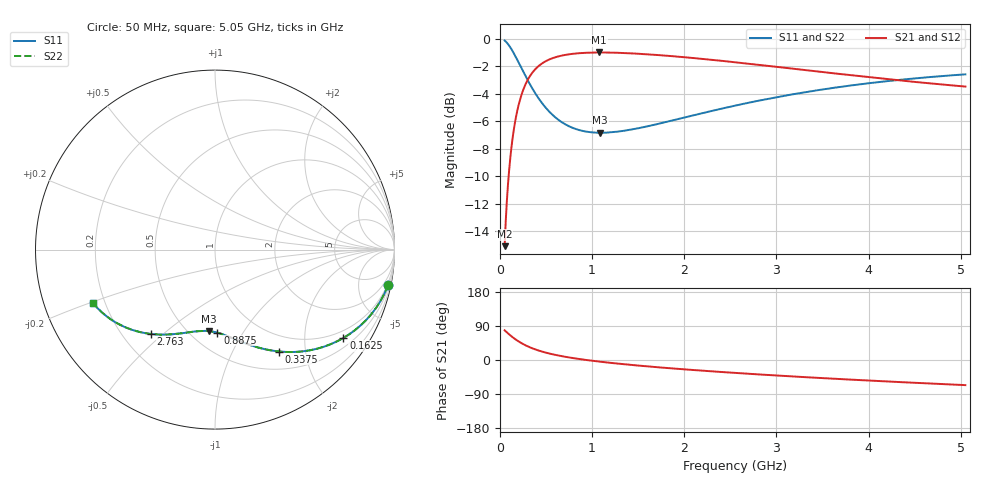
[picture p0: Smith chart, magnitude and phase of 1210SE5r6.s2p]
! AVX Thin Film Operation		Date: August 2001
! Description: Accu-P® Series, Thin Film, SMD, RF Capacitor
! Part Number: 1210J5R6ABT
! 50 MHz  -  5.05 GHz
! Serial Measurements
# mhz S db R 50
!	S11		S21		S12		S22
!	dB	Phase	dB	Phase	dB	Phase	dB	Phase
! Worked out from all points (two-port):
!   401 points, 50 MHz to 5.05 GHz, reference 50 ohm
!   highest |S21| = -1.01 dB at 1.075 GHz (marker M1); lowest = -15.1 dB at 50 MHz (marker M2)
!   |S21| within 3 dB of the highest: 236.8 MHz to end of sweep
!   lowest |S11| = -6.8 dB at 1.087 GHz (marker M3), VSWR 2.67, Z = 31 - j35.5 ohm
!   |S11| at or under -10 dB: nowhere
!   |S22| runs from -6.8 to -0.1 dB; largest |S21 - S12| = 0
!   S11 on the Smith chart (normalised r, x): 50 MHz: 0.76, -9.75; 162.5 MHz: 0.76, -3.05; 337.5 MHz: 0.75, -1.54; 887.5 MHz: 0.66, -0.78; 2.763 GHz: 0.31, -0.45; 5.05 GHz: 0.15, -0.21
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50  -0.14 -11.6  -15.07 78.4  -15.07 78.4  -0.14 -11.6
75  -0.30 -17.2  -11.74 72.8  -11.74 72.8  -0.30 -17.2
87.5  -0.41 -19.9  -10.52 70.1  -10.52 70.1  -0.41 -19.9
112.5  -0.65 -25.1  -8.61 64.9  -8.61 64.9  -0.65 -25.1
162.5  -1.23 -34.5  -6.09 55.5  -6.09 55.5  -1.23 -34.5
200  -1.71 -40.7  -4.88 49.3  -4.88 49.3  -1.71 -40.7
237.5  -2.21 -46.2  -4.00 43.8  -4.00 43.8  -2.21 -46.2
337.5  -3.47 -57.8  -2.60 32.2  -2.60 32.2  -3.47 -57.8
437.5  -4.52 -66.4  -1.90 23.6  -1.90 23.6  -4.52 -66.4
562.5  -5.49 -74.4  -1.44 15.5  -1.44 15.5  -5.49 -74.4
712.5  -6.24 -81.7  -1.18 8.3  -1.18 8.3  -6.24 -81.7
887.5  -6.69 -88.3  -1.05 1.6  -1.05 1.6  -6.69 -88.3
1075  -6.84 -94.1  -1.01 -4.2  -1.01 -4.2  -6.84 -94.1
1087.5  -6.84 -94.5  -1.01 -4.5  -1.01 -4.5  -6.84 -94.5
1400  -6.63 -102.4  -1.06 -12.4  -1.06 -12.4  -6.63 -102.4
1725  -6.18 -109.4  -1.20 -19.4  -1.20 -19.4  -6.18 -109.4
2125  -5.53 -116.9  -1.43 -26.9  -1.43 -26.9  -5.53 -116.9
2550  -4.87 -124.0  -1.72 -34.1  -1.72 -34.1  -4.87 -124.0
2762.5  -4.57 -127.3  -1.87 -37.4  -1.87 -37.4  -4.57 -127.3
3387.5  -3.81 -136.3  -2.34 -46.3  -2.34 -46.3  -3.81 -136.3
4225  -3.07 -146.9  -2.96 -56.9  -2.96 -56.9  -3.08 -146.9
5050  -2.60 -156.3  -3.48 -66.3  -3.48 -66.3  -2.60 -156.3
